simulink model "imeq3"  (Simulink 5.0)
settings: Solver=ode45  StartTime=0.0  StopTime=1  MaxStep=0.002  RelTol=1e-3
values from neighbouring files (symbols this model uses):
  den = cosh(2*q)-cos(2*q)    [imbar1.m]    (also in imbarB.m; imdef0vec.m = 0.91; imdef1vec.m = 0.91; imic2.m = Lm*Lsl+Lm*Lrl+Lsl*Lrl)
  Hi = str2num(get(h,'string'))    [imic33.m]
  ic = [fs0 fr0]    [imdef0vec.m]    (also in imdef1vec.m; imdef2vec.m = F; imic2.m = [phids phiqs phidr phiqr n0]'; imic3.m = [phids phiqs phidr phiqr n0]')
  Lm = eval(get(hLm,'String'))    [im3d.m]    (also in IMabc2.m = 4.5; imabcparam.m = 0.0847; IMabcrun0.m = 0.0847; IMabcrun1.m = 0.0847)
  Lrl = eval(get(hLr,'String'))    [im3d.m]    (also in IMabc2.m = 0.1; imabcparam.m = 0.0025; IMabcrun0.m = 0.0025; IMabcrun1.m = 0.0025)
  Lsl = eval(get(hLs,'String'))    [im3d.m]    (also in IMabc2.m = 0.1; imabcparam.m = 0.0025; IMabcrun0.m = 0.0025; IMabcrun1.m = 0.0025)
  Rr = input('Rotor resistance)[default = 2] =')    [Actac.m]    (also in im1phase.m = 0.3; im3d.m = eval(get(hRr,'String')); IMabc2.m = 0.02; imabcparam.m = 0.408)
  Rs = eval(get(hRs,'String'))    [im3d.m]    (also in IMabc2.m = 0.01; imabcparam.m = 0.531; IMabcrun0.m = 0.531; IMabcrun1.m = 0.531)
  Tl0 = Is*conj(Is)*Req    [imdef0vec.m]    (also in imdef1vec.m; imdef2vec.m = Lm*(I(2)*I(3)-I(1)*I(4)); imdefrotflux.m; imdefSIvec1.m = Te0/To)
  vs = 1.0    (= 1)    [imdef0vec.m]    (also in imdef1vec.m; imdef2vec.m; imdefrotflux.m; imdefSIvec1.m)
  wk = ws    (= 1)    [imdef0vec.m]    (also in imdef1vec.m; imdef2vec.m; imdefrotflux.m; imdefSIvec1.m)
  wo = 2*pi*freq0    [calc0.m]    (also in IMabc2.m = 376.991118431; imabcparam.m = 376.991118431; IMabcrun0.m = 376.991118431; IMabcrun1.m = 376.991118431)

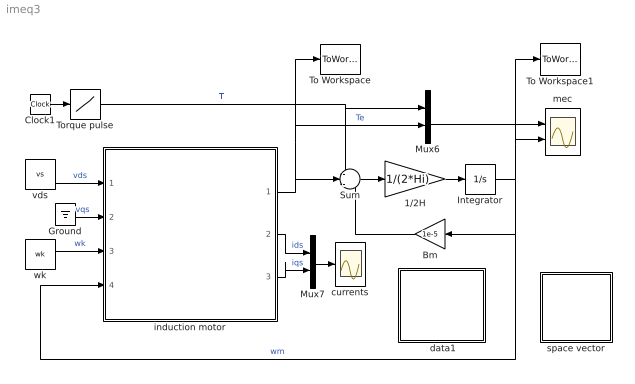
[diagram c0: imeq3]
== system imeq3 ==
  " data1" : Subsystem
  1/2H : Gain  Gain=1/(2*Hi)
  Bm : Gain  Orientation=left  Gain=1e-5
  Clock1 : Clock
  Ground : Ground
  Integrator : Integrator  InitialCondition=ic(5)
  Mux6 : Mux  Inputs=2
  Mux7 : Mux  Inputs=2
  Sum : Sum  Inputs=-+-
  To Workspace : ToWorkspace  VariableName=Te  SampleTime=-1  SaveFormat=Array
  To Workspace1 : ToWorkspace  VariableName=wm  SampleTime=-1  SaveFormat=Array
  Torque pulse : Lookup  InputValues=[0 0.1 0.1 0.5 0.5 2]  OutputValues="[Tl0 Tl0  0 0 0.5 0.5]"
  currents : Scope
  induction motor : Subsystem
  mec : Scope  NumInputPorts=2
  space vector : Subsystem
  vds : Constant  Value=vs
  wk : Constant  Value=wk
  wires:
  vds/1 -> induction motor/1(vds)  "vds"
  Ground/1 -> induction motor/2(vqs)  "vqs"
  wk/1 -> induction motor/3(wk)  "wk"
  Sum/1 -> 1/2H/1
  1/2H/1 -> Integrator/1
  Bm/1 -> Sum/3
  induction motor/1(Te) -> Sum/2, Mux6/2, To Workspace/1  "Te"
  Integrator/1 -> Bm/1, induction motor/4(wm), mec/2, To Workspace1/1  "wm"
  Mux6/1 -> mec/1
  Mux7/1 -> currents/1
  induction motor/2(ids) -> Mux7/1  "ids"
  induction motor/3(iqs) -> Mux7/2  "iqs"
  Clock1/1 -> Torque pulse/1
  Torque pulse/1 -> Mux6/1, Sum/1  "Tl"

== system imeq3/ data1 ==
  note: This demo simulates the running of an induction motor in steady-state when a sudden input change is effected: a)torque step changes at constant voltage excitation b) voltage input sag at constant frequency and load torque c)simultaneous step changes in voltage magnitude and frequency
  note: Double click the block to enter the machine parameters and initial conditions and then run the simulation

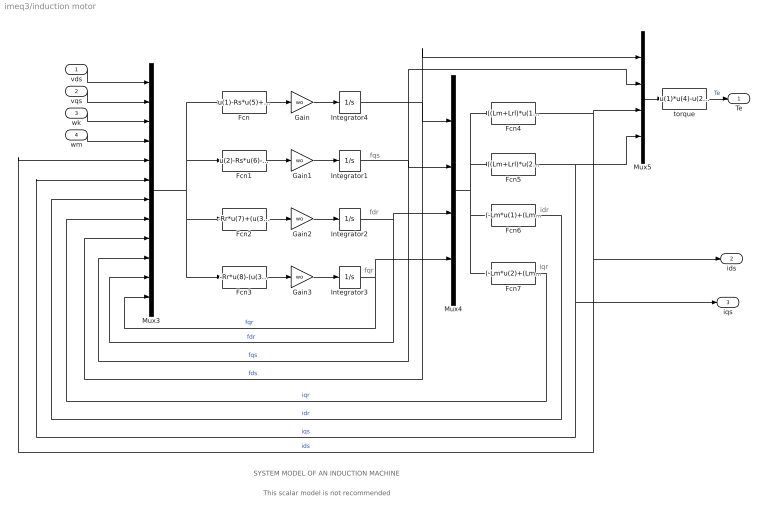
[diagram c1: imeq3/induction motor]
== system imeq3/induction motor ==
  note: fqs
  note: fdr
  note: fqr
  note: SYSTEM MODEL OF AN INDUCTION MACHINE
  note: This scalar model is not recommended
  note: idr
  note: iqr
  vds : Inport
  vqs : Inport  Port=2
  wk : Inport  Port=3
  wm : Inport  Port=4
  Fcn : Fcn  Expr=u(1)-Rs*u(5)+u(3)*u(10)
  Fcn1 : Fcn  Expr=u(2)-Rs*u(6)-u(3)*u(9)
  Fcn2 : Fcn  Expr=-Rr*u(7)+(u(3)-u(4))*u(12)
  Fcn3 : Fcn  Expr=-Rr*u(8)-(u(3)-u(4))*u(11)
  Fcn4 : Fcn  Expr=((Lm+Lrl)*u(1)-Lm*u(3))/den
  Fcn5 : Fcn  Expr=((Lm+Lrl)*u(2)-Lm*u(4))/den
  Fcn6 : Fcn  Expr=(-Lm*u(1)+(Lm+Lsl)*u(3))/den
  Fcn7 : Fcn  Expr=(-Lm*u(2)+(Lm+Lsl)*u(4))/den
  Gain{,1..3} (4 alike) : Gain  Gain=wo
  Integrator1 : Integrator  InitialCondition=ic(2)
  Integrator2 : Integrator  InitialCondition=ic(3)
  Integrator3 : Integrator  InitialCondition=ic(4)
  Integrator4 : Integrator  InitialCondition=ic(1)
  Mux3 : Mux  Inputs=12
  Mux4 : Mux
  Mux5 : Mux
  torque : Fcn  Expr=u(1)*u(4)-u(2)*u(3)
  Te : Outport
  ids : Outport  Port=2
  iqs : Outport  Port=3
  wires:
  Fcn1/1 -> Gain1/1
  Gain1/1 -> Integrator1/1
  Mux3/1 -> Fcn1/1, Fcn/1, Fcn3/1, Fcn2/1
  Fcn2/1 -> Gain2/1
  Gain2/1 -> Integrator2/1
  Fcn/1 -> Gain/1
  Gain/1 -> Integrator4/1
  Integrator3/1 -> Mux4/4, Mux3/12  "fqr"
  Integrator2/1 -> Mux4/3, Mux3/11  "fdr"
  Integrator1/1 -> Mux3/10, Mux4/2, Mux5/2  "fqs"
  Integrator4/1 -> Mux4/1, Mux3/9, Mux5/1  "fds"
  Fcn7/1 -> Mux3/8  "iqr"
  Fcn6/1 -> Mux3/7  "idr"
  Fcn3/1 -> Gain3/1
  Gain3/1 -> Integrator3/1
  Mux4/1 -> Fcn4/1, Fcn5/1, Fcn7/1, Fcn6/1
  Fcn5/1 -> Mux5/4, Mux3/6, iqs/1  "iqs"
  Fcn4/1 -> Mux5/3, Mux3/5, ids/1  "ids"
  Mux5/1 -> torque/1
  vds/1 -> Mux3/1
  vqs/1 -> Mux3/2
  wk/1 -> Mux3/3
  wm/1 -> Mux3/4
  torque/1 -> Te/1  "Te"

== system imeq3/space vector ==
